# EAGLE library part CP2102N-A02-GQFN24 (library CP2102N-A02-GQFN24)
USB Interface IC USB to UART bridge - QFN24 Source: Datasheet Check availability
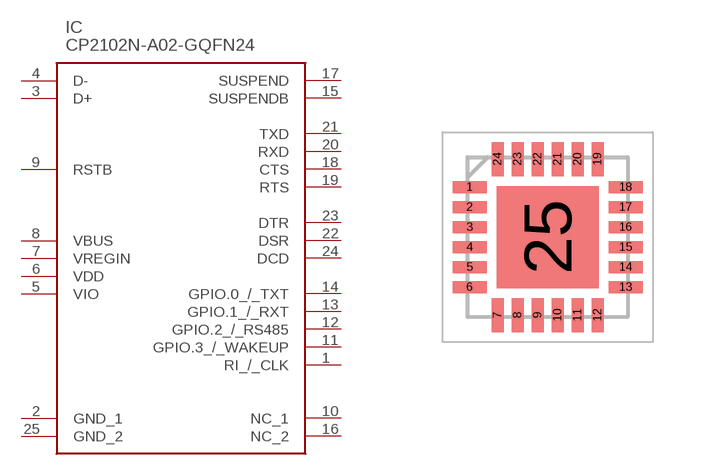
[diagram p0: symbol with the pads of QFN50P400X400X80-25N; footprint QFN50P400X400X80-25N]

Designator prefix IC

## CP2102N-A02-GQFN24 (Availability: In Stock; Description: USB Bridge, USB to UART USB 2.0 UART Interface 24-QFN (4x4); MF: Silicon Labs; MP: CP2102N-A02-GQFN24; Package: WFQFN-24 Silicon Labs; Price: None; Purchase-URL: https://pricing.snapeda.com/search/part/CP2102N-A02-GQFN24/?ref=eda)  [QFN50P400X400X80-25N]
1  RI_/_CLK
2  GND_1  pwr
3  D+
4  D-
5  VIO  pwr
6  VDD  pwr
7  VREGIN  pwr
8  VBUS  pwr
9  RSTB
10  NC_1  nc
11  GPIO.3_/_WAKEUP
12  GPIO.2_/_RS485
13  GPIO.1_/_RXT
14  GPIO.0_/_TXT
15  SUSPENDB  out
16  NC_2  nc
17  SUSPEND  out
18  CTS
19  RTS  out
20  RXD  in
21  TXD  out
22  DSR
23  DTR
24  DCD
25  GND_2  pwr

## Footprint QFN50P400X400X80-25N (pad centres in mm)
QFN24 *
smd 0.85 x 0.3: 1 -1.95,1.25; 2 -1.95,0.75; 3 -1.95,0.25; 4 -1.95,-0.25; 5 -1.95,-0.75; 6 -1.95,-1.25; 13 1.95,-1.25; 14 1.95,-0.75; 15 1.95,-0.25; 16 1.95,0.25; 17 1.95,0.75; 18 1.95,1.25
smd 0.3 x 0.85: 7 -1.25,-1.95; 8 -0.75,-1.95; 9 -0.25,-1.95; 10 0.25,-1.95; 11 0.75,-1.95; 12 1.25,-1.95; 19 1.25,1.95; 20 0.75,1.95; 21 0.25,1.95; 22 -0.25,1.95; 23 -0.75,1.95; 24 -1.25,1.95
smd 2.55 x 2.55: 25 0,0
